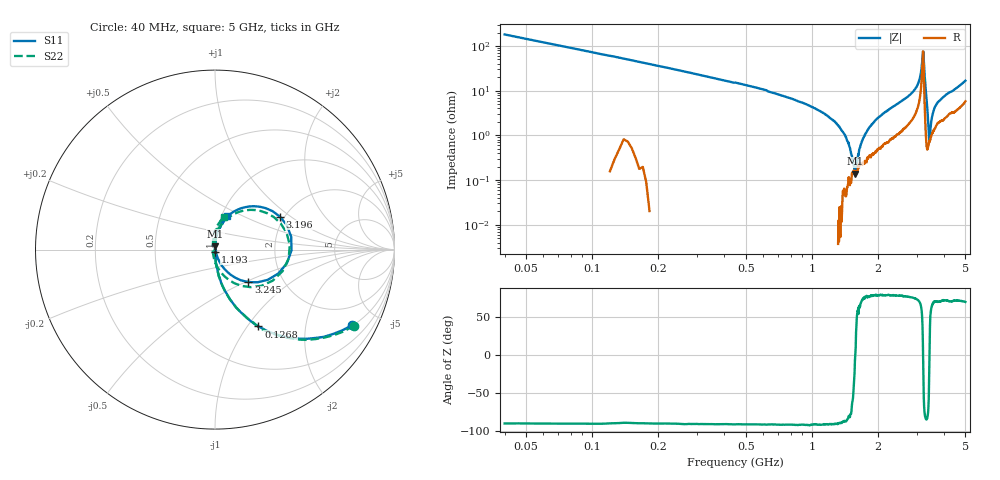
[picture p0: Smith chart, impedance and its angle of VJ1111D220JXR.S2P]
! VJ1111D220JXR
! DATE 02/16/2022  10:15
! CAPACITORS MOUNTED IN SERIES ON 25 MIL THICK MICROSTRIP SUBSTRATE
# GHz  S  MA  R  50.00
!  FREQ  S11M  S11A  S21M  S21A  S12M  S12A  S22M  S22A
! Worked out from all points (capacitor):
!   801 points, 40 MHz to 5 GHz, reference 50 ohm
!   read as one part in series: C = 21.8 pF near 64.8 MHz
!   lowest |Z| = 138 mohm at 1.571 GHz (marker M1)
!   series resonance near 1.576 GHz, so ESL is about 470 pH
!   S11 on the Smith chart (normalised r, x): 40 MHz: 1.02, -3.60; 126.8 MHz: 1.00, -1.13; 1.193 GHz: 1.00, -0.02; 3.196 GHz: 1.90, +0.83; 3.245 GHz: 1.34, -0.52; 5 GHz: 1.06, +0.41
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0.04  0.8723 -29.0  0.4844 61.2  0.4826 60.9  0.883 -28.7
0.1268  0.4913 -60.6  0.8597 29.3  0.8817 30.3  0.4984 -60.4
0.3066  0.2197 -77.5  0.9764 13.1  0.982 12.9  0.2208 -77.6
0.8708  0.04691 -87.0  0.9992 3.9  1.003 3.8  0.04686 -87.9
1.1932  0.01161 -89.1  0.9974 2.5  1.004 2.3  0.01113 -91.7
1.2614  0.005419 -81.4  0.9975 2.2  1.003 2.0  0.005554 -101.3
1.3048  0.002015 -77.5  0.9969 2.0  1.003 1.8  0.001271 -111.9
1.3234  0.0002456 -1.3  0.9971 2.0  1.002 1.8  0.0001307 150.8
1.3668  0.004271 82.7  0.9971 1.8  1.002 1.6  0.004025 100.3
1.3978  0.006231 83.1  0.9963 1.7  1.002 1.5  0.006225 95.2
1.5714  0.0193 86.6  0.995 1.2  1.001 1.1  0.01957 91.4
1.6954  0.02839 87.2  0.9935 0.9  0.9993 0.7  0.02826 89.3
2.52  0.08359 82.9  0.9777 -1.2  0.9835 -1.4  0.08361 84.7
3.0718  0.1826 71.4  0.9259 -6.0  0.9305 -6.1  0.1784 69.7
3.1958  0.406 26.9  0.6218 -8.5  0.6249 -8.5  0.3941 21.7
3.2454  0.2595 -44.2  0.8521 18.2  0.8575 18.0  0.2511 -53.7
3.3508  0.005204 -36.7  0.9833 4.7  0.9883 4.6  0.01367 -156.6
3.3694  0.01082 73.2  0.9823 3.9  0.9876 3.9  0.0153 150.7
3.4376  0.04218 88.7  0.9782 2.2  0.9837 2.0  0.03977 106.4
3.5554  0.07208 87.2  0.9692 0.8  0.9757 0.6  0.06508 97.3
4.1754  0.1327 77.4  0.9531 -2.0  0.9583 -2.1  0.1147 82.6
5  0.1969 70.2  0.9121 -5.6  0.9173 -5.8  0.1858 74.5
